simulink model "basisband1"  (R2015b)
settings: Solver=VariableStepAuto  StartTime=0.0  StopTime=10.0  RelTol=1e-3
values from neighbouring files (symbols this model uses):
  delta_f1 = 200    [basisband_1.m]    (also in basisband_2.m)
  delta_f2 = 250    [basisband_1.m]    (also in basisband_2.m = 300)
  f0 = 5000    [basisband_1.m]    (also in basisband_2.m = 40000; mehrdeutigkeit_1.m = 200; spektr_pulse_1.m = 1010)
  Ts = 1/fs    (= 5e-05)    [basisband_1.m]    (also in basisband_2.m = 5e-06; dezimier_1.m = 0.0005; dezimier_11.m = 0.0005; dezimier_2.m = 0.0005)
undefined symbols (not defined in the file or in its folder): fir1
libraries: simulink x1, dspsrcs4 x1

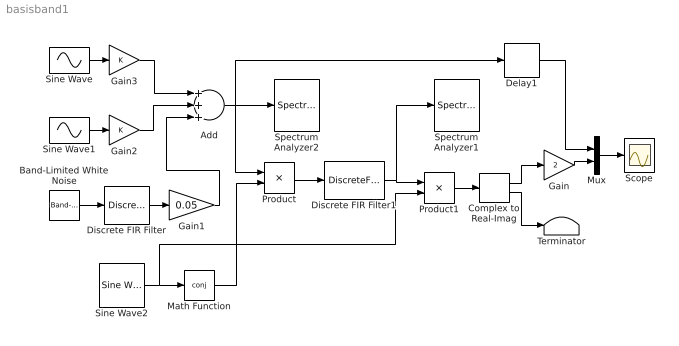
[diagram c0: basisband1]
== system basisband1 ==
  Add : Sum  Inputs=+++
  Band-Limited White Noise : simulink/Sources/Band-Limited White Noise  Cov=Ts  Ts=Ts  seed=[23341]
  Complex to Real-Imag : ComplexToRealImag
  Delay1 : Delay  DelayLength=128
  Discrete FIR Filter : DiscreteFir  Coefficients=fir1(128, [0.1, 0.3])
  Discrete FIR Filter1 : DiscreteFir  Coefficients=fir1(256, 0.1)
  Gain : Gain  Gain=2
  Gain1 : Gain  Gain=0.05
  Gain2 : Gain
  Gain3 : Gain
  Math Function : Math  Operator=conj
  Mux : Mux  Inputs=2
  Product : Product
  Product1 : Product
  Scope : Scope
  Sine Wave : Sin  Frequency=2*pi*(f0+delta_f1)  SampleTime=Ts
  Sine Wave1 : Sin  Amplitude=0.5  Frequency=2*pi*(f0-delta_f2)  SampleTime=Ts
  Sine Wave2 : dspsrcs4/Sine Wave  Amplitude=1  Frequency=f0  Phase=0  SampleMode=Discrete  OutComplex=Complex  CompMethod=Trigonometric fcn  TableSize=Speed  SampleTime=Ts  SamplesPerFrame=1  ResetState=Restart at time zero  OutputFrames=off  dataType=double  wordLen=16  udDataType=sfix(16)  fracBitsMode=Best precision  numFracBits=15  OutDataTypeStr=double  LastOutDataTypeStr=double
  Spectrum Analyzer1 : SpectrumAnalyzer
  Spectrum Analyzer2 : SpectrumAnalyzer
  Terminator : Terminator
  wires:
  Sine Wave/1 -> Gain3/1
  Sine Wave1/1 -> Gain2/1
  Math Function/1 -> Product/2
  Product/1 -> Discrete FIR Filter1/1
  Sine Wave2/1 -> Product1/2, Math Function/1
  Product1/1 -> Complex to Real-Imag/1
  Gain/1 -> Mux/2
  Add/1 -> Spectrum Analyzer2/1, Product/1, Delay1/1
  Mux/1 -> Scope/1
  Band-Limited White Noise/1 -> Discrete FIR Filter/1
  Discrete FIR Filter/1 -> Gain1/1
  Gain1/1 -> Add/3
  Complex to Real-Imag/1 -> Gain/1
  Complex to Real-Imag/2 -> Terminator/1
  Discrete FIR Filter1/1 -> Product1/1, Spectrum Analyzer1/1
  Delay1/1 -> Mux/1
  Gain2/1 -> Add/2
  Gain3/1 -> Add/1
